(* Logix 5000 AddOnInstructionDefinition export CFW900_2171; software revision 20.06 *)

ADD_ON_INSTRUCTION CFW900_2171   (* revision 1.0, ExecutePrescan *)
// 21/71 CIP Extended Speed
// AOI
// Help:
// Drive setup as follows:
// C9.5.1 = 21/71
// C4.1.1 - Ethernet
// C4.2.2.1 - Ethernet
// C4.2.2.2 - Ethernet
// C4.2.2.3 - Ethernet
// C4.2.2.4 - Ethernet
// C4.3.1.2.1 - Keypad
// C4.3.1.2.2 - Ethernet
VAR_INPUT
   ConnectionFaulted : BOOL; {required}   // From CFW900
END_VAR
VAR_IN_OUT
   Inputs : INT[2]; {required}   // Input Assembly From CFW900
   Outputs : INT[2]; {required}   // Output Assembly To CFW900
END_VAR
VAR_INPUT
   Run_Fwd : BOOL; {visible}   // 1 = Run Fwd 0 = Stop
   Run_Rev : BOOL; {visible}   // 1 = Run Rev 0 = Stop
   Fault_Reset : BOOL; {visible}   // 1 = Fault Reset 0 = No action
   NetCtrl : BOOL := 1; {visible}   // 1 = Remote (PLC) Control 0 = Local (HMI) Control
   NetRef : BOOL := 1; {visible}   // 1 = Speed Reference is sent via network 0 = Speed Reference is not being sent via network
   Speed_Reference : INT; {required}   // Speed Setpoint (RPM)
END_VAR
VAR_OUTPUT
   RealSpeed : INT; {access Read Only, visible}   // Current Speed (RPM)
   Connection_Ready : BOOL; {access None, visible}   // Indicates that CFW900 connection is not in a faulted state
   Connection_Faulted : BOOL; {access Read Only, visible}   // Connection is interrupted status bit
   sts_Drv_nrdy : BOOL; {access None, visible}   // 1 = Drive not ready latched until no run cmd given
   Faulted : BOOL; {access Read Only, visible}
   Running_Fwd : BOOL; {access Read Only, visible}   // 1 = CFW900 Running 0 = CFW900 Stopped
   Running_Rev : BOOL; {access Read Only, visible}   // 1 = Motor is rotating 0 = Motor is not rotating
   Warning : BOOL; {access Read Only, visible}   // 1 = drive is in alarm condition 0 = drive is not in alarm condition
   Ready : BOOL; {access Read Only, visible}   // 1 = Drive is ready to operate (states Ready, Enabled or Stopping) 0 = Drive is not ready to operate
   Ctrl_from_net : BOOL; {access Read Only, visible}   // 1 = drive is controlled remotely (PLC) 0 = drive is controlled locally (HMI)
   Ref_from_net : BOOL; {access Read Only, visible}   // 1 = using speed/torque reference received via network 0 = speed/torque reference received via network is disregarded
   At_reference : BOOL; {access Read Only, visible}   // 1 = drive has reached the programmed speed 0 = drive has not yet reached the programmed speed
END_VAR
VAR_INPUT
   cfg_FailToStartDelay : DINT; {access None, visible}
   cfg_FailToStopDelay : DINT; {access None, visible}
END_VAR
VAR_OUTPUT
   FailedToStart : BOOL; {access Read Only, visible}   // Indicates Drive Failed to Start
   FailedToStop : BOOL; {access None, visible}   // Indicates Drive Failed to stop in the time allotted
   Drive_Status : INT; {access Read Only, visible}   // 0 = Non-Existent 1= Startup 2 = Not Ready 3 = Ready 4 = Enabled 5 = Stopping 6 = Fault Stop 7 = Faulted
END_VAR
VAR
   FailToStart : TIMER; {access None}
   Wrk_Run1 : BOOL; {access None}   // Internal bit to signal run1
   Wrk_Run2 : BOOL; {access None}   // Internal bit to signal run2
   FailToStop : TIMER; {access None}
END_VAR

ROUTINE Logic   (* ladder *)
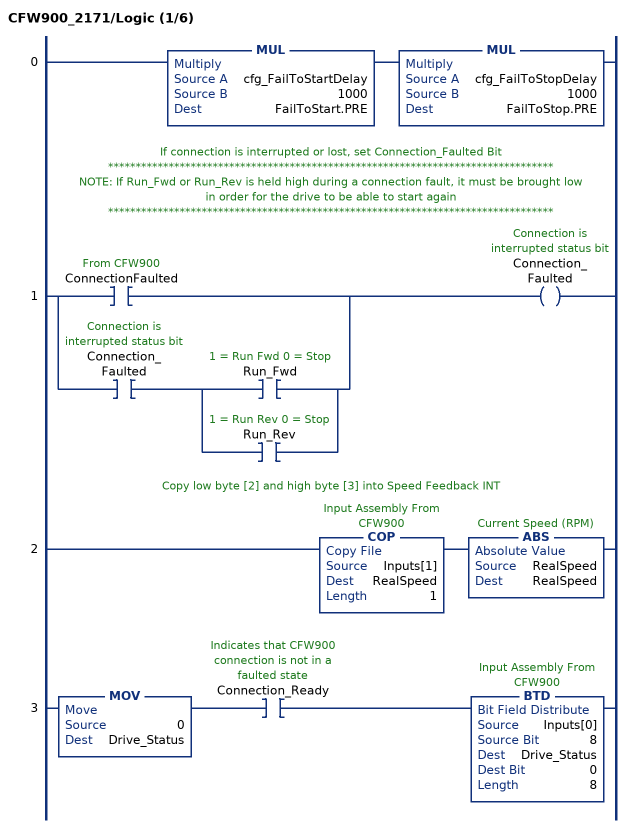
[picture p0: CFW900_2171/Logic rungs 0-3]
   0: MUL(cfg_FailToStartDelay,1000,FailToStart.PRE)MUL(cfg_FailToStopDelay,1000,FailToStop.PRE);
   // If connection is interrupted or lost, set Connection_Faulted Bit
   // *********************************************************************************
   // NOTE: If Run_Fwd or Run_Rev is held high during a connection fault, it must be brought low
   // in order for the drive to be able to start again
   // *********************************************************************************
   1: [XIC(ConnectionFaulted) ,XIC(Connection_Faulted) [XIC(Run_Fwd) ,XIC(Run_Rev) ] ]OTE(Connection_Faulted);
   // Copy low byte [2] and high byte [3] into Speed Feedback INT
   2: COP(Inputs[1],RealSpeed,1)ABS(RealSpeed,RealSpeed);
   3: MOV(0,Drive_Status)XIC(Connection_Ready)BTD(Inputs[0],8,Drive_Status,0,8);
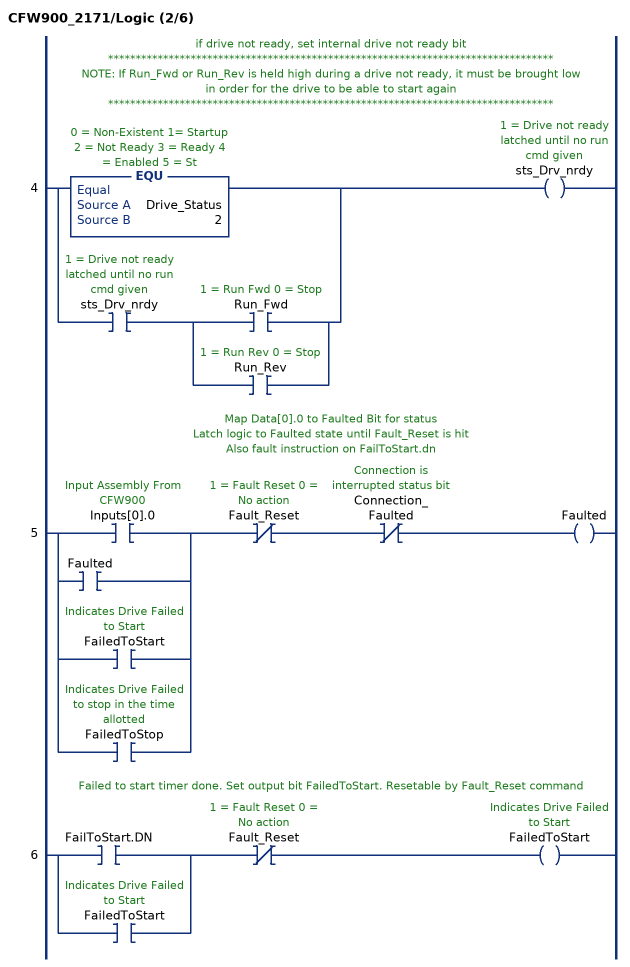
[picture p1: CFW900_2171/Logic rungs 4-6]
   // if drive not ready, set internal drive not ready bit
   // *********************************************************************************
   // NOTE: If Run_Fwd or Run_Rev is held high during a drive not ready, it must be brought low
   // in order for the drive to be able to start again
   // *********************************************************************************
   4: [EQU(Drive_Status,2) ,XIC(sts_Drv_nrdy) [XIC(Run_Fwd) ,XIC(Run_Rev) ] ]OTE(sts_Drv_nrdy);
   // Map Data[0].0 to Faulted Bit for status
   // Latch logic to Faulted state until Fault_Reset is hit
   // Also fault instruction on FailToStart.dn
   5: [XIC(Inputs[0].0) ,XIC(Faulted) ,XIC(FailedToStart) ,XIC(FailedToStop) ]XIO(Fault_Reset)XIO(Connection_Faulted)OTE(Faulted);
   // Failed to start timer done. Set output bit FailedToStart. Resetable by Fault_Reset command
   6: [XIC(FailToStart.DN) ,XIC(FailedToStart) ]XIO(Fault_Reset)OTE(FailedToStart);
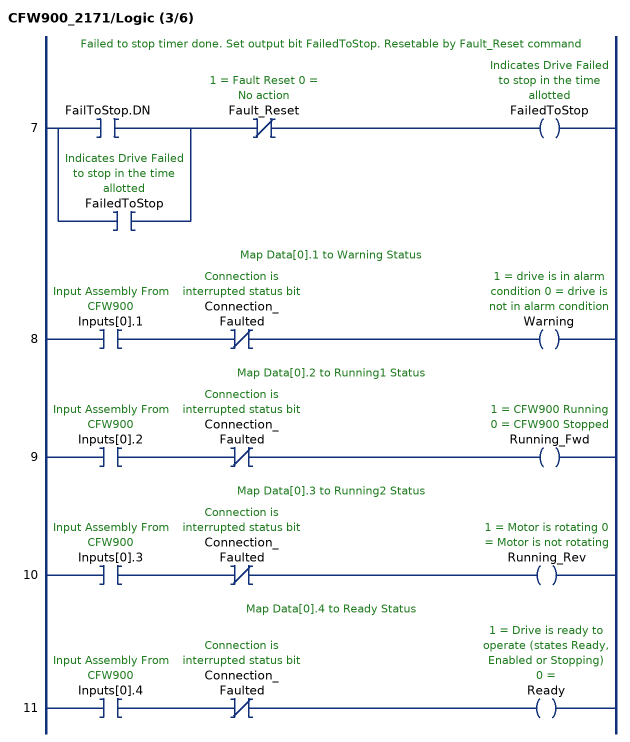
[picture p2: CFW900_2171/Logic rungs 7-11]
   // Failed to stop timer done. Set output bit FailedToStop. Resetable by Fault_Reset command
   7: [XIC(FailToStop.DN) ,XIC(FailedToStop) ]XIO(Fault_Reset)OTE(FailedToStop);
   // Map Data[0].1 to Warning Status
   8: XIC(Inputs[0].1)XIO(Connection_Faulted)OTE(Warning);
   // Map Data[0].2 to Running1 Status
   9: XIC(Inputs[0].2)XIO(Connection_Faulted)OTE(Running_Fwd);
   // Map Data[0].3 to Running2 Status
   10: XIC(Inputs[0].3)XIO(Connection_Faulted)OTE(Running_Rev);
   // Map Data[0].4 to Ready Status
   11: XIC(Inputs[0].4)XIO(Connection_Faulted)OTE(Ready);
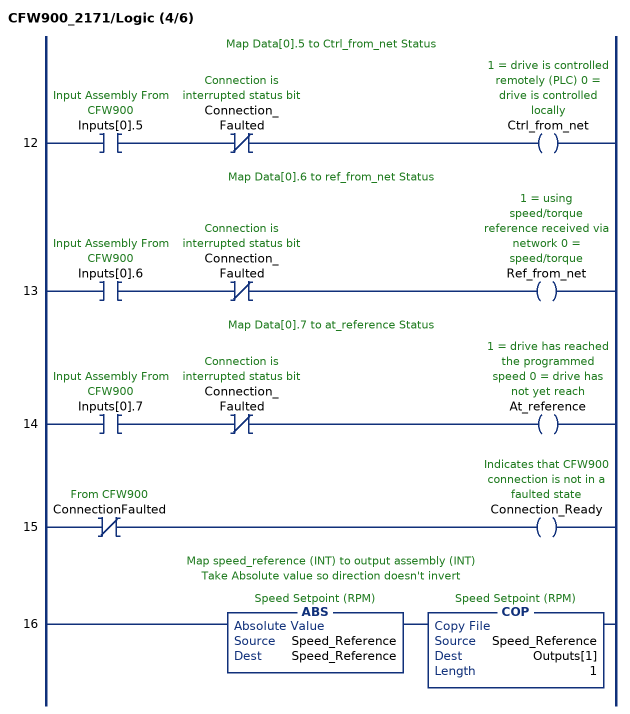
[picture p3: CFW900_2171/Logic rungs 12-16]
   // Map Data[0].5 to Ctrl_from_net Status
   12: XIC(Inputs[0].5)XIO(Connection_Faulted)OTE(Ctrl_from_net);
   // Map Data[0].6 to ref_from_net Status
   13: XIC(Inputs[0].6)XIO(Connection_Faulted)OTE(Ref_from_net);
   // Map Data[0].7 to at_reference Status
   14: XIC(Inputs[0].7)XIO(Connection_Faulted)OTE(At_reference);
   15: XIO(ConnectionFaulted)OTE(Connection_Ready);
   // Map speed_reference (INT) to output assembly (INT)
   // Take Absolute value so direction doesn't invert
   16: ABS(Speed_Reference,Speed_Reference)COP(Speed_Reference,Outputs[1],1);
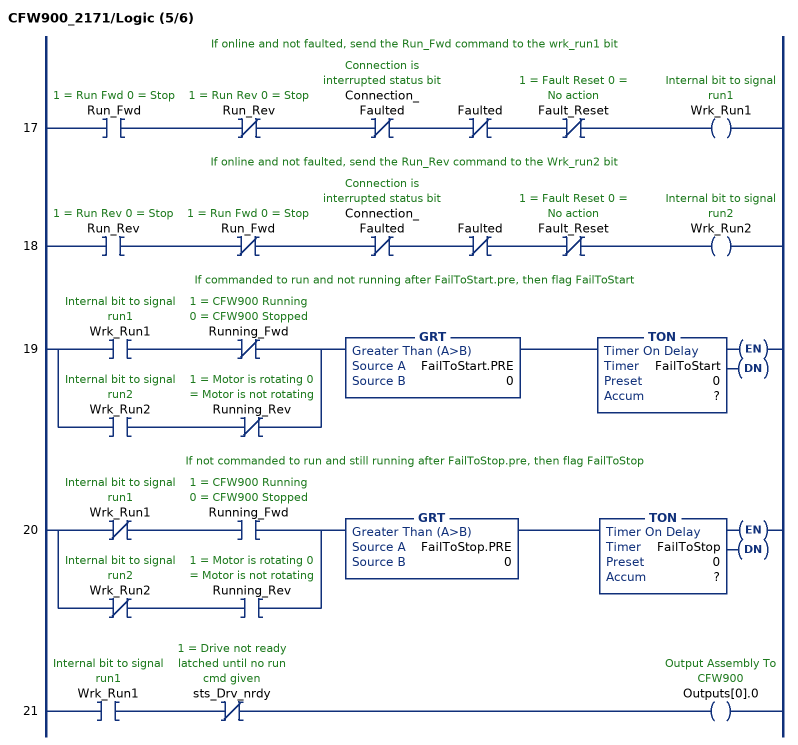
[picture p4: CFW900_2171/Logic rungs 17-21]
   // If online and not faulted, send the Run_Fwd command to the wrk_run1 bit
   17: XIC(Run_Fwd)XIO(Run_Rev)XIO(Connection_Faulted)XIO(Faulted)XIO(Fault_Reset)OTE(Wrk_Run1);
   // If online and not faulted, send the Run_Rev command to the Wrk_run2 bit
   18: XIC(Run_Rev)XIO(Run_Fwd)XIO(Connection_Faulted)XIO(Faulted)XIO(Fault_Reset)OTE(Wrk_Run2);
   // If commanded to run and not running after FailToStart.pre, then flag FailToStart
   19: [XIC(Wrk_Run1) XIO(Running_Fwd) ,XIC(Wrk_Run2) XIO(Running_Rev) ]GRT(FailToStart.PRE,0)TON(FailToStart,?,?);
   // If not commanded to run and still running after FailToStop.pre, then flag FailToStop
   20: [XIO(Wrk_Run1) XIC(Running_Fwd) ,XIO(Wrk_Run2) XIC(Running_Rev) ]GRT(FailToStop.PRE,0)TON(FailToStop,?,?);
   21: XIC(Wrk_Run1)XIO(sts_Drv_nrdy)OTE(Outputs[0].0);
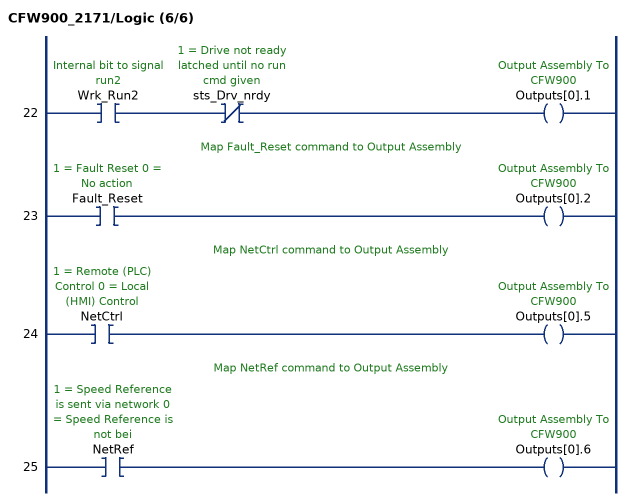
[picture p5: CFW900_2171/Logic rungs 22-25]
   22: XIC(Wrk_Run2)XIO(sts_Drv_nrdy)OTE(Outputs[0].1);
   // Map Fault_Reset command to Output Assembly
   23: XIC(Fault_Reset)OTE(Outputs[0].2);
   // Map NetCtrl command to Output Assembly
   24: XIC(NetCtrl)OTE(Outputs[0].5);
   // Map NetRef command to Output Assembly
   25: XIC(NetRef)OTE(Outputs[0].6);
END_ROUTINE

ROUTINE Prescan   (* ladder *)
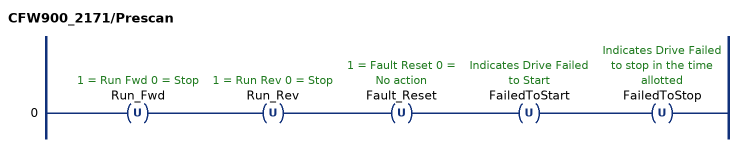
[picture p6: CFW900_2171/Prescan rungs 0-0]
   0: OTU(Run_Fwd)OTU(Run_Rev)OTU(Fault_Reset)OTU(FailedToStart)OTU(FailedToStop);
END_ROUTINE
END_ADD_ON_INSTRUCTION
